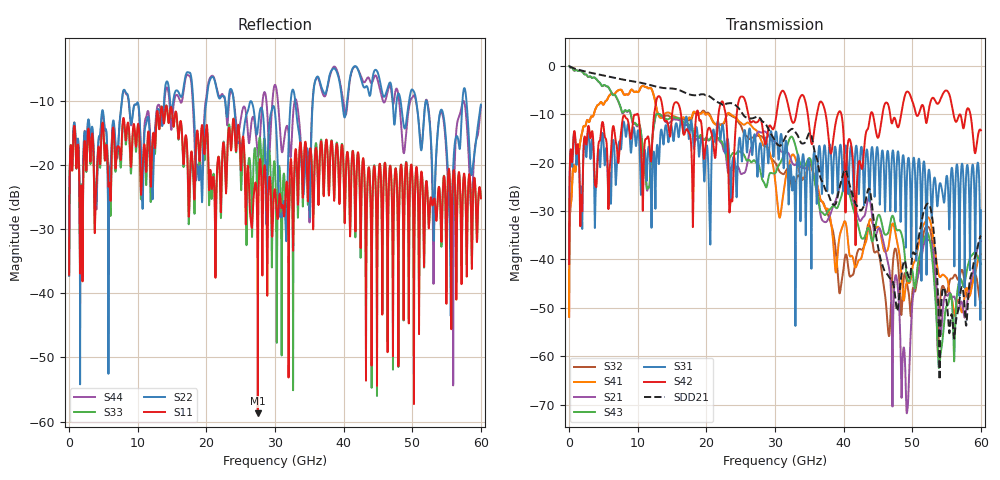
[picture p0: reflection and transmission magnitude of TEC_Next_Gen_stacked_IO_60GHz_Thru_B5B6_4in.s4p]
!! CHANNEL DESCRIPTION:  Next Generation 28Gbps Press-fit Stacked I/O Connector
!!  with 4" 5-6-5 Megtron 6 Stripline trace on host side and 1.25" 7-5-7 Megtron 6 Microstrip trace on plug side
!! HOST PCB DESCRIPTION:  PCB thickness 3.425 mm
!!  26 Layer Board, 15 GND planes, 4 Layer route-out on Layers 7,11,17,21, 8mil stub on vias
!!  Pairs on following layers
!!  Layer 07 - A02A03 A14A15 D05D06
!!  Layer 11 - D020D3 C05C06 D14D15
!!  Layer 17 - C02C03 B05B06 C14C15
!!  Layer 21 - B02B03 A05A06 B14B15
!! CONNECTOR DESCRIPTION:  Next Generation 28Gbps Press-fit Stacked I/O Connector
!! PLUG-IN CARD DESCRIPTION:  PCB thickness 1mm thick
!!  6 Layer Board, 4 GND planes, 0.35 x 1.4mm mating pads
!!  Micro-strip diff traces referenced to GND plane 3mils down, 2nd GND plane 17mils from top of board
!!  PCB GND planes are symmetric
!! MODEL DESCRIPTION: TE Connectivity S-parameter model produced from Macro-model, Extracted .s4p THRU (PAIR B05B06)
!! MODEL DATE: 5/15/2014 CR32f, FPR23
!! MODEL STATUS: Developmental
!! MODEL GEOMETRY: 4 Rows - Rows A, B, C, D. 3 pairs in each row, 12 total pairs
!! MODEL FREQUENCY RANGE: DC to 60 GHz in 10 MHz frequency steps
!! MODEL EDGE RATE LIMITATION: 8.33 ps (Using conservative 0.5/Fmax rule of thumb)
!! TIME-DOMAIN TRANSFORM CAUTIONS:
!! 1.) Do not simulate transient edge rates faster than the number listed above.  Edge
!!  rates faster than this number contain significant spectral content at frequencies
!!  above the model's highest frequency.
!! 2.) Even when simulating edge rates that are slower than the number listed above, be
!!  aware that the best time resolution possible with a direct iFFT is (1 / 2Fmax).
!!  As a result, time resolution is typically not adequate for most time-domain
!!  simulations unless tricks such as frequency-domain zero-padding and windowing are
!!  used to minimize leakage and aliasing.
!! 3.) Because the model has a uniform frequency step, a direct iFFT will result in an
!!  impulse that that has a time length given by either (1 / Fstep) or (1 / 2Fstep),
!!  depending on the transform being used.  Care has been taken in selecting the
!!  frequency step to ensure a settled impulse response for the model.  Therefore,
!!  convolution with the model's impulse response should present no issues.  However,
!!  if directly concatenating s-parameter models in the frequency domain a user must
!!  either interpolate necessary interim frequencies or complete impulse response
!!  zero-padding.  Impulse response zero-padding is more difficult, but more accurate.
!! PORT DEFINITIONS:
!! Port  1  ----->  Host B05		B05 Module <-----  Port  2
!! Port  3  ----->  Host B06		B06 Module <-----  Port  4
! Touchstone data
! Created: 29-Sep-2014 by IdEM R2011 (7.0.3)
# Hz S MA R 50
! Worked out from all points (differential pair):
!   6000 points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, 10 MHz to 60 GHz, reference 50 ohm
!   strongest paths, dB at 10 MHz, 15.01 GHz, 30.01 GHz, 45.01 GHz, 60 GHz:
!     S42: -41.0, -10.1, -12.0, -14.9, -13.4
!     S31: -40.9, -13.2, -14.6, -17.9, -29.9
!     S43: -0.1, -10.7, -22.2, -31.0, -40.9
!     S21: -0.1, -11.3, -15.7, -33.8, -36.3
!     S41: -51.9, -10.2, -23.5, -33.3, -38.9
!     S32: -51.9, -10.8, -20.0, -38.5, -49.0
!   taken as a pair (ports 3,1 in; 4,2 out), SDD21 dB: -0.1, -4.7, -15.5, -37.3, -35.1
!   lowest |S11| = -58.7 dB at 27.49 GHz (marker M1), VSWR 1.00, Z = 49.9 + j0.1 ohm
!   |S11| at or under -10 dB: start of sweep to end of sweep
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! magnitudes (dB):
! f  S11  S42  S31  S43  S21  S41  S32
! 10 MHz  -37.1  -41.0  -40.9  -0.1  -0.1  -51.9  -51.9
! 6.03 GHz  -25.5  -19.6  -25.1  -5.1  -5.1  -5.9  -5.9
! 27.49 GHz  -58.7  -11.6  -22.5  -20.3  -13.7  -13.7  -14.4
! 43.75 GHz  -20.9  -11.5  -27.9  -33.9  -27.5  -32.1  -32.9
! 49.27 GHz  -21.5  -5.3  -21.5  -44.1  -71.4  -44.8  -45.3
! 51.89 GHz  -25.1  -10.7  -22.9  -35.2  -36.0  -32.3  -33.5
! 60 GHz  -25.2  -13.4  -29.9  -40.9  -36.3  -38.9  -49.0
